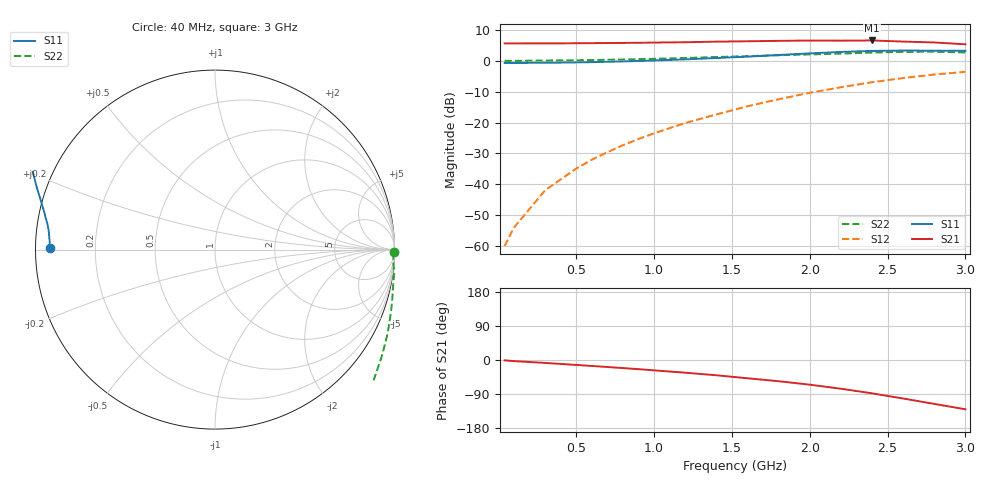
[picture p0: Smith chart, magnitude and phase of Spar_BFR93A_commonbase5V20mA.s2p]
! Filename:  BFR93ACC.S2P  Version:  2.0
! NXP part #: BFR93A  Date: Jul 1990
! Bias condition: Vce=5V, Ic=20mA
! COMMON BASE
#  MHz  S  MA  R  50
! Freq  S11  S21  S12  S22
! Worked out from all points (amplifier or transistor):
!   21 points, 40 MHz to 3 GHz, reference 50 ohm
!   highest |S21| = 6.5 dB at 2.4 GHz (marker M1)
!   |S21| within 3 dB of that: start of sweep to end of sweep
!   unconditionally stable (mu >= 1): nowhere
!   at 300 MHz: K = -0.68, MSG = 23.8 dB, |S12| = -41.9 dB
!   at 1 GHz: K = -0.94, MSG = 14.7 dB, |S12| = -23.5 dB
!   at 3 GHz: K = -0.83, MSG = 4.4 dB, |S12| = -3.6 dB
40  0.922 179.4  1.905 -0.9  0.001 45.4  0.996 -0.9
100  0.921 178.2  1.904 -2.9  0.002 84.9  0.994 -2.7
200  0.923 176.8  1.907 -5.3  0.004 113.5  0.999 -5.0
300  0.927 175.4  1.906 -7.7  0.008 127.4  1.007 -7.5
400  0.931 173.9  1.906 -10.3  0.012 133.9  1.01 -10.1
500  0.938 172.4  1.915 -13.1  0.018 139.1  1.016 -12.8
600  0.947 170.9  1.922 -15.7  0.025 141.2  1.025 -15.5
700  0.961 169.3  1.932 -18.5  0.033 142.6  1.035 -18.2
800  0.973 167.7  1.938 -21.3  0.043 144.2  1.046 -21.0
900  0.99 166.0  1.947 -24.2  0.054 145.1  1.058 -23.7
1000  1.008 164.3  1.963 -27.3  0.067 144.6  1.073 -26.7
1200  1.051 160.8  1.988 -33.5  0.098 143.5  1.105 -32.9
1400  1.104 156.9  2.032 -40.3  0.135 140.8  1.145 -39.5
1600  1.162 152.5  2.06 -48.2  0.183 137.8  1.186 -46.6
1800  1.236 147.4  2.092 -56.0  0.238 133.0  1.224 -54.6
2000  1.312 142.0  2.118 -65.1  0.302 127.7  1.262 -63.7
2200  1.386 136.2  2.107 -75.8  0.372 121.4  1.3 -74.5
2400  1.438 129.0  2.124 -87.9  0.448 113.6  1.352 -86.0
2600  1.46 120.7  2.037 -101.6  0.524 105.4  1.388 -97.6
2800  1.453 111.0  1.971 -115.9  0.597 96.1  1.396 -109.4
3000  1.445 101.4  1.84 -130.0  0.661 88.2  1.359 -120.9
